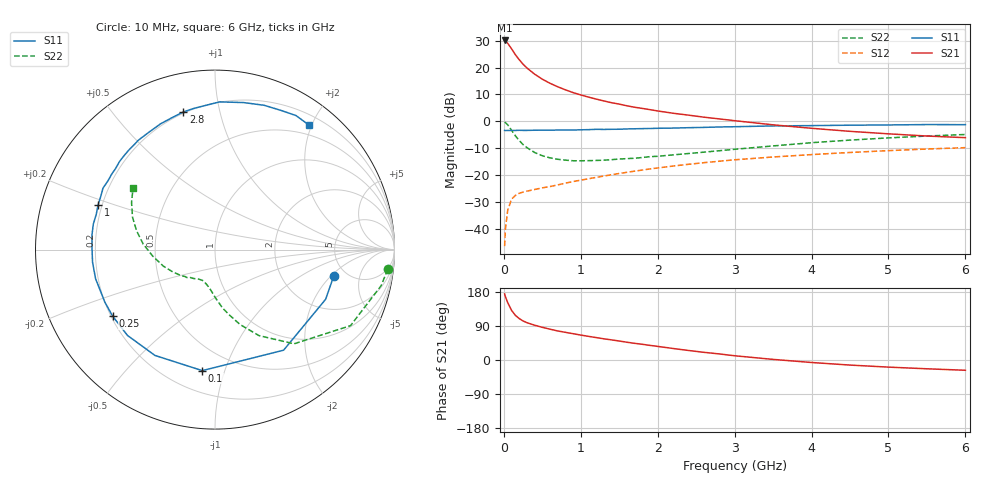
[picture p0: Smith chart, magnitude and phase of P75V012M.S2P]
! SIEMENS Small Signal Semiconductors
! BFP196
! Si NPN RF Bipolar Junction Transistor in SOT143
! VCE = 5 V  IC = 12 mA
! Common Emitter S-Parameters:  May  1996
# GHz  S  MA  R  50
!  f  S11  S21  S12  S22
! GHz  MAG  ANG  MAG  ANG  MAG  ANG  MAG  ANG
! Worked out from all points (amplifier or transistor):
!   36 points, 10 MHz to 6 GHz, reference 50 ohm
!   highest |S21| = 30.1 dB at 10 MHz (marker M1)
!   |S21| within 3 dB of that: start of sweep to 97.85 MHz
!   unconditionally stable (mu >= 1): 842 MHz to 3.243 GHz
!   at 250 MHz: K = 0.44, MSG = 23.8 dB, |S12| = -26.3 dB
!   at 1.4 GHz: K = 1.13, MAG = 11.2 dB, |S12| = -19.8 dB
!   at 6 GHz: K = 0.96, MSG = 1.9 dB, |S12| = -9.8 dB
!   S11 on the Smith chart (normalised r, x): 10 MHz: 4.01, -2.15; 100 MHz: 0.34, -0.84; 250 MHz: 0.21, -0.29; 1 GHz: 0.18, +0.18; 2.8 GHz: 0.19, +0.78; 6 GHz: 0.34, +1.95
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0.01  0.6782 -12.3  31.89 174.5  0.0048 83.6  0.9686 -6.5
0.02  0.6757 -24.2  30.93 167.3  0.0099 79.4  0.947 -12.3
0.05  0.6784 -55.7  28.29 151.3  0.0222 65.4  0.8658 -29.3
0.1  0.678 -96.0  22.35 131.1  0.0359 50.3  0.6852 -50.0
0.15  0.678 -119.6  17.35 117.8  0.0421 41.9  0.5384 -62.9
0.2  0.683 -135.6  14.01 109.3  0.046 37.5  0.4414 -71.4
0.25  0.6801 -146.9  11.54 103.0  0.0486 35.7  0.3706 -77.9
0.3  0.68 -154.5  9.83 98.5  0.0506 35.7  0.3257 -82.9
0.4  0.6848 -166.3  7.55 91.8  0.0542 35.3  0.2643 -90.1
0.5  0.6859 -174.2  6.075 86.2  0.0582 37.3  0.2301 -95.3
0.6  0.6856 178.9  5.103 81.3  0.0615 39.1  0.2098 -100.1
0.7  0.6904 173.1  4.399 76.7  0.0661 40.7  0.1976 -104.3
0.8  0.6927 168.1  3.857 73.0  0.0711 42.0  0.1905 -107.8
1  0.6974 159.0  3.1 65.8  0.0809 43.9  0.1852 -113.0
1.1  0.7023 155.0  2.826 62.4  0.0859 44.9  0.1865 -115.9
1.6  0.7238 137.3  1.947 46.9  0.1132 45.8  0.2033 -128.7
2.2  0.7506 119.3  1.417 30.4  0.148 42.8  0.2386 -142.5
2.8  0.787 103.0  1.112 16.0  0.1819 37.5  0.2846 -157.9
3.5  0.8234 88.2  0.863 1.6  0.2179 29.8  0.35 -174.3
4.5  0.8494 71.2  0.653 -13.4  0.2645 19.0  0.4489 166.6
5.5  0.8725 58.9  0.534 -23.2  0.3064 7.9  0.5342 150.5
6  0.8694 53.1  0.498 -27.1  0.3252 1.8  0.5711 143.1
